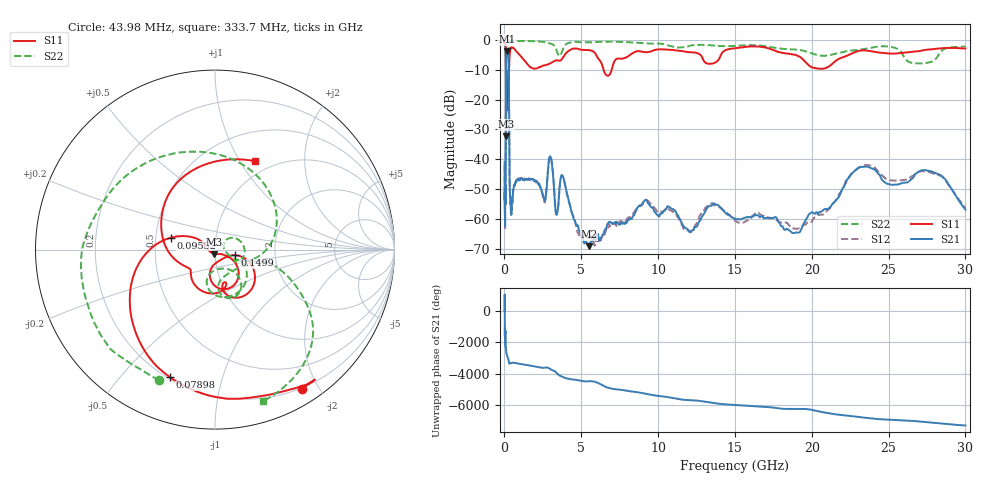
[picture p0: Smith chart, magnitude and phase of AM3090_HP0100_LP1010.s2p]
! Date/Time: Thu, Feb 28, 2019 1:57 PM
! Network Analyzer: Agilent Technologies E8364B Rev: A.07.50.67
! Sweep from 0.010 to 30.000 GHz, 1601 Points, Sweep Type: LOG
! Power Supply: 5.023 V, 0.002 A
# Hz S DB R 50
!freq MagS11 AngS11 MagS21 AngS21 MagS12 AngS12 MagS22 AngS22
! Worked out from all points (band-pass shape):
!   1601 points, 10 MHz to 30 GHz, reference 50 ohm
!   highest |S21| = -3.85 dB at 154.4 MHz (marker M1); lowest = -69.2 dB at 5.501 GHz (marker M2)
!   |S21| within 3 dB of the highest: 106.2 MHz to 270.8 MHz (164.7 MHz wide, 87.3 % of centre)
!   lowest |S11| = -32.3 dB at 104 MHz (marker M3), VSWR 1.05, Z = 49.5 - j2.36 ohm
!   |S11| at or under -10 dB: 94.42 MHz to 297.9 MHz (203.4 MHz wide, 104 % of centre); 6.454 GHz to 6.978 GHz (523.7 MHz wide, 7.8 % of centre)
!   |S22| runs from -26.2 to -0.2 dB; largest |S21 - S12| = 0.015
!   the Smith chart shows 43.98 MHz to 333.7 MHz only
!   S11 on the Smith chart (normalised r, x): 43.98 MHz: 0.19, -1.79; 78.98 MHz: 0.21, -0.69; 95.52 MHz: 0.60, +0.09; 149.9 MHz: 1.24, -0.08; 333.7 MHz: 0.84, +1.16
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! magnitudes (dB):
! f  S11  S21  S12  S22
! 10 MHz  -0.3  -41.0  -42.1  -0.6
! 38.04 MHz  -0.5  -61.4  -57.7  -1.6
! 43.98 MHz  -0.8  -60.6  -58.7  -2.0
! 78.98 MHz  -2.5  -49.1  -48.1  -4.7
! 95.52 MHz  -11.9  -15.7  -15.6  -11.5
! 104 MHz  -32.3  -7.6  -7.6  -25.7
! 119.1 MHz  -13.0  -5.1  -5.0  -17.0
! 144.7 MHz  -23.1  -4.0  -3.9  -17.9
! 149.9 MHz  -18.9  -3.9  -3.9  -17.2
! 154.4 MHz  -15.4  -3.9  -3.8  -15.9
! 274.6 MHz  -14.7  -7.4  -7.4  -16.2
! 333.7 MHz  -5.3  -48.0  -47.1  -1.1
! 550.5 MHz  -2.7  -51.6  -52.0  -0.3
! 2.084 GHz  -9.6  -47.2  -47.6  -0.4
! 2.987 GHz  -7.8  -39.0  -39.0  -1.2
! 3.385 GHz  -6.8  -58.7  -58.4  -3.4
! 3.798 GHz  -6.0  -45.7  -45.7  -3.2
! 5.501 GHz  -3.4  -69.2  -66.6  -0.8
! 7.926 GHz  -5.8  -61.4  -60.4  -0.7
! 18.74 GHz  -4.8  -64.8  -63.3  -3.2
! 23.36 GHz  -3.5  -42.5  -42.3  -3.1
! 30 GHz  -2.8  -56.9  -56.3  -2.2
